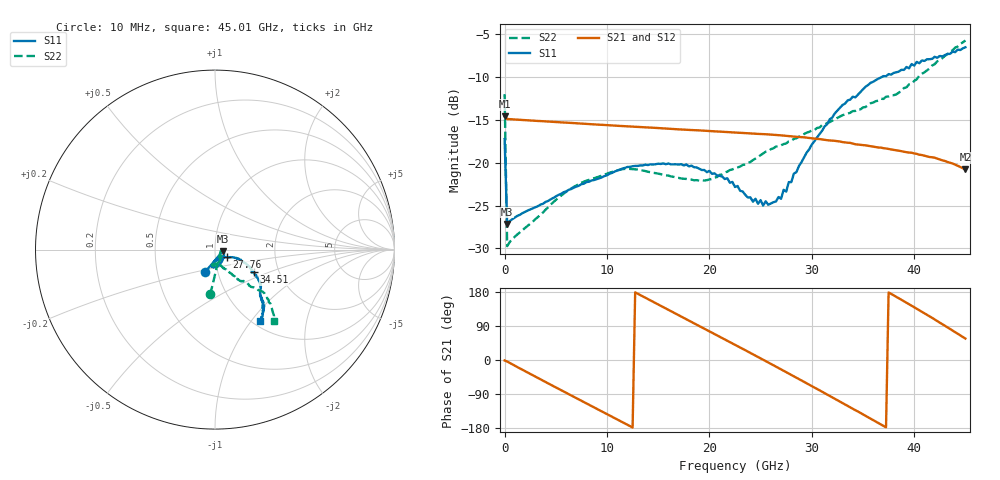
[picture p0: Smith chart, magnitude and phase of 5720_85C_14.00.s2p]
! Device:  ADRF5720
! Description: 0.5dB LSB GaAs MMIC 6-bit Digital Attenuator
! Frequency:  0.000009 -  40 GHz
! Ports:
!	RF1	= Port 1
!	RF2	= Port 2
! Vdd:  3.3 Volt
! Vss:  -3.3 Volt
! Control:  0/3.3 Volt
! State:  14.00 dB attenuation
! Data:  The device was measured using G-S-G Probes on a matrix board.
!  Data was collected using an calibrated 4 port network analyzer.
!  The reference plane for this measurement is at the launchers.
! Note:  Analog Devices supplies this data as a sample of measured data
!  for this product.  Your particular data for this product may vary.
!  Data was taken at 85 degrees C.
!  Analog Devices reserves the right to change this data at anytime.
# GHZ S DB R 45.0
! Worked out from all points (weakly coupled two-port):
!   181 points, 10 MHz to 45.01 GHz, reference 45 ohm
!   highest |S21| = -14.59 dB at 10 MHz (marker M1); lowest = -20.8 dB at 45.01 GHz (marker M2)
!   lowest |S11| = -27.1 dB at 260 MHz (marker M3), VSWR 1.09, Z = 49 - j0.853 ohm
!   |S11| at or under -10 dB: start of sweep to 36.82 GHz
!   |S22| runs from -29.7 to -5.7 dB; largest |S21 - S12| = 0.00089
!   S11 on the Smith chart (normalised r, x): 10 MHz: 0.87, -0.22; 27.76 GHz: 1.13, -0.10; 34.51 GHz: 1.49, -0.39; 45.01 GHz: 1.08, -1.11
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0.01  -17.24 -113.8  -14.59 -1.3  -14.57 -1.3  -11.99 -96.0
0.26  -27.15 -11.4  -14.89 -4.0  -14.88 -4.0  -29.74 -15.0
4.26  -24.46 -35.6  -15.19 -61.6  -15.17 -61.6  -25.20 -52.6
7.76  -22.44 -58.8  -15.44 -111.2  -15.43 -111.1  -22.21 -77.0
11.51  -20.68 -78.5  -15.71 -163.9  -15.71 -163.8  -20.74 -93.8
15.26  -20.14 -92.4  -15.96 143.1  -15.95 143.2  -21.33 -99.7
19.01  -20.69 -99.6  -16.22 90.1  -16.21 90.2  -22.09 -88.3
22.76  -22.71 -94.3  -16.49 36.7  -16.47 36.9  -20.55 -71.5
25.26  -25.00 -74.2  -16.66 0.8  -16.64 1.0  -18.91 -65.2
27.01  -24.21 -44.3  -16.80 -24.8  -16.78 -24.5  -17.95 -60.7
27.26  -23.16 -39.4  -16.83 -28.4  -16.82 -28.2  -17.82 -60.9
27.51  -23.37 -37.3  -16.86 -32.1  -16.85 -31.8  -17.74 -59.6
27.76  -22.26 -33.3  -16.88 -35.7  -16.87 -35.5  -17.51 -60.2
28.01  -22.26 -33.0  -16.92 -39.5  -16.90 -39.2  -17.43 -59.3
28.26  -21.27 -29.0  -16.94 -43.0  -16.93 -42.8  -17.22 -59.7
30.26  -17.49 -23.1  -17.18 -72.5  -17.16 -72.2  -16.20 -56.8
33.01  -13.26 -26.6  -17.59 -113.6  -17.57 -113.3  -14.45 -53.5
34.51  -12.06 -29.8  -17.87 -135.8  -17.85 -135.6  -13.73 -52.8
35.76  -10.66 -34.5  -18.06 -154.9  -18.05 -154.7  -13.05 -51.5
37.76  -9.71 -39.4  -18.46 174.5  -18.44 174.8  -12.11 -46.8
41.51  -7.91 -48.6  -19.33 115.2  -19.30 115.6  -9.00 -41.4
45.01  -6.52 -57.9  -20.78 56.6  -20.74 57.0  -5.72 -50.5
